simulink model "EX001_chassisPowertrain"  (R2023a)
settings: Solver=ode23tb  StartTime=0.0  StopTime=20e3  MaxStep=1e-1  RelTol=1e-4
libraries: component_lib x8, slpidlib x1

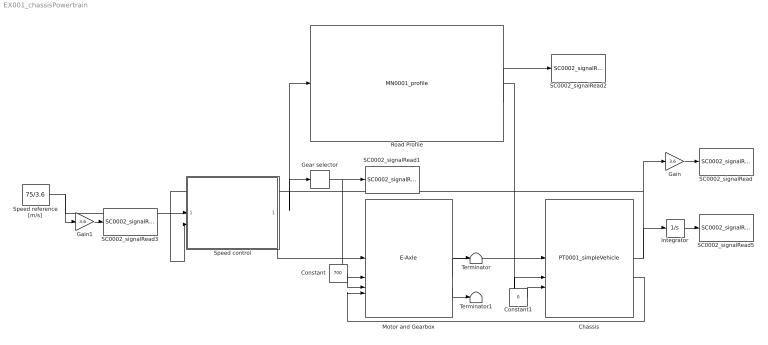
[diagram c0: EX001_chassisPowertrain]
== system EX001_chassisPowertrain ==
  Chassis : component_lib/Powertrain/PT0001_simpleVehicle  m=40e3  r_w=0.5  A_f=10  C_d=0.5  rho_air=1.225  c_r0=0.0060  c_r1=2.3e-7  gain=600  v0=75/3.6  x0=0
  Constant : Constant  Value=700
  Constant1 : Constant  Value=0
  Gain : Gain  Gain=3.6
  Gain1 : Gain  Gain=3.6
  Gear selector : Relay  OnSwitchValue=22  OffSwitchValue=21.5  OnOutputValue=4  OffOutputValue=3
  Integrator : Integrator
  Motor and Gearbox : component_lib/E-Axle  n=3  V_nom=700
  Road Profile : component_lib/Mission/MN0001_profile  profile=Munchen.mat  x0=0  N_lookahead=100
  SC0002_signalRead : component_lib/Data & Control/SC0002_signalRead  SigName=velocity
  SC0002_signalRead1 : component_lib/Data & Control/SC0002_signalRead  SigName=gear
  SC0002_signalRead2 : component_lib/Data & Control/SC0002_signalRead  SigName=altitude
  SC0002_signalRead3 : component_lib/Data & Control/SC0002_signalRead  SigName=velocityReference
  SC0002_signalRead5 : component_lib/Data & Control/SC0002_signalRead  SigName=distance
  Speed control : Subsystem
  Speed reference [m/s] : Constant  Value=75/3.6
  Terminator : Terminator
  Terminator1 : Terminator
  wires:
  Motor and Gearbox/1 -> Chassis/1
  Motor and Gearbox/2 -> Terminator/1
  Motor and Gearbox/3 -> Terminator1/1
  Chassis/2 -> Motor and Gearbox/4
  Road Profile/1 -> Chassis/2
  Chassis/1 -> Integrator/1, Gain/1, Speed control/2(v [m/s]), Road Profile/1, Gear selector/1
  Speed reference [m/s]/1 -> Gain1/1, Speed control/1(v_ref [m/s])
  Speed control/1(Tq_sig [-]) -> Motor and Gearbox/1
  Gear selector/1 -> Motor and Gearbox/2, SC0002_signalRead1/1
  Integrator/1 -> SC0002_signalRead5/1
  Gain/1 -> SC0002_signalRead/1
  Road Profile/2 -> SC0002_signalRead2/1
  Gain1/1 -> SC0002_signalRead3/1
  Constant/1 -> Motor and Gearbox/3
  Constant1/1 -> Chassis/3

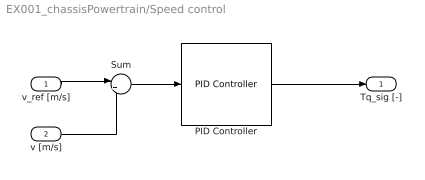
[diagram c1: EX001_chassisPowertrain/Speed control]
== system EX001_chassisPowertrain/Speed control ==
  v_ref [m/s] : Inport
  v [m/s] : Inport  Port=2
  PID Controller : slpidlib/PID Controller  Controller=PID  Form=Parallel  TimeDomain=Continuous-time  UseExternalTs=off  SampleTime=-1  IntegratorMethod=Forward Euler  FilterMethod=Forward Euler  ControllerParametersSource=internal  P=10  I=1e-1  UseKiTs=off  D=0  N=100  UseFilter=on  TunerSelectOption=Transfer Function Based (PID Tuner App)  ZeroCross=off  InitialConditionSource=internal  InitialConditionForIntegrator=0  InitialConditionForFilter=0  DifferentiatorICPrevScaledInput=0  ExternalReset=none  TrackingMode=off  Kt=1  LimitOutput=on  SatLimitsSource=internal  UpperSaturationLimit=1  LowerSaturationLimit=-1  LinearizeAsGain=on  AntiWindupMode=clamping  Kb=1  LimitIntegrator=off  UpperIntegratorSaturationLimit=inf  LowerIntegratorSaturationLimit=-inf  POutMin=[]  POutMax=[]  IOutMin=[]  IOutMax=[]  DOutMin=[]  DOutMax=[]  NOutMin=[]  NOutMax=[]  SumOutMin=[]  SumOutMax=[]  SaturationOutMin=[]  SaturationOutMax=[]  PParamMin=[]  PParamMax=[]  IParamMin=[]  IParamMax=[]  DParamMin=[]  DParamMax=[]  NParamMin=[]  NParamMax=[]  KbParamMin=[]  KbParamMax=[]  KtParamMin=[]  KtParamMax=[]  KbOutMin=[]  KbOutMax=[]  KtOutMin=[]  KtOutMax=[]  IntegratorOutMin=[]  IntegratorOutMax=[]  FilterOutMin=[]  FilterOutMax=[]  SumI1OutMin=[]  SumI1OutMax=[]  SumI2OutMin=[]  SumI2OutMax=[]  SumI3OutMin=[]  SumI3OutMax=[]  SumI4OutMin=[]  SumI4OutMax=[]  SumDOutMin=[]  SumDOutMax=[]  DifferentiatorOutMin=[]  DifferentiatorOutMax=[]  FilterDiffOutCoefMin=[]  FilterDiffOutCoefMax=[]  ReciprocalOutMin=[]  ReciprocalOutMax=[]  SumDenOutMin=[]  SumDenOutMax=[]  SumNumOutMin=[]  SumNumOutMax=[]  DivideOutMin=[]  DivideOutMax=[]  UdiffTsProdOutMin=[]  UdiffTsProdOutMax=[]  NTsProdOutMin=[]  NTsProdOutMax=[]  UintegralTsProdOutMin=[]  UintegralTsProdOutMax=[]  UngainTsProdOutMin=[]  UngainTsProdOutMax=[]  ClampingZeroOutDataTypeStr=Inherit: Inherit via back propagation  ClampingZeroOutMin=[]  ClampingZeroOutMax=[]  FilterDenConstantOutDataTypeStr=Inherit: Inherit via back propagation  FilterDenConstantOutMin=[]  FilterDenConstantOutMax=[]  PCopyOutDataTypeStr=Inherit: Inherit via back propagation  PCopyOutMin=[]  PCopyOutMax=[]  NCopyOutDataTypeStr=Inherit: Inherit via back propagation  NCopyOutMin=[]  NCopyOutMax=[]  IntegratorContinuousStateAttributes=''  IntegratorStateMustResolveToSignalObject=off  IntegratorRTWStateStorageClass=Auto  FilterContinuousStateAttributes=''  FilterStateMustResolveToSignalObject=off  FilterRTWStateStorageClass=Auto  ParallelPVariant=InternalParameters  IdealPVariant=Disabled  IVariant=InternalParameters  DVariant=InternalParameters  IntegratorVariant=Continuous  SatVariant=Enabled  AWVariant=ContClampingParallel  PCopyVariant=Disabled  TRVariant=Disabled  FdbkBlocksVariant=Forward  IdealPFdbkVariant=Disabled  SatFdbkVariant=Disabled  DerivativeFilterVariant=ContFilter  NVariant=InternalParameters  NCopyVariant=Disabled  FilterICVariant=InternalICsFilter  IntegratorICVariant=InternalICs  ExternalResetVariant=Disabled  TRSumVariant=Passthrough  SumFdbkVariant=Disabled  SumVariant=Sum_PID  TsampFilterVariant=InternalTs  TsampNgainVariant=Passthrough  TsampIntegralVariant=Disabled_SignalSpec  ExternalSaturationOutDataTypeStr=Inherit: Same as second input
  Sum : Sum  Inputs=|+-
  Tq_sig [-] : Outport
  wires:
  PID Controller/1 -> Tq_sig [-]/1
  Sum/1 -> PID Controller/1
  v_ref [m/s]/1 -> Sum/1
  v [m/s]/1 -> Sum/2
